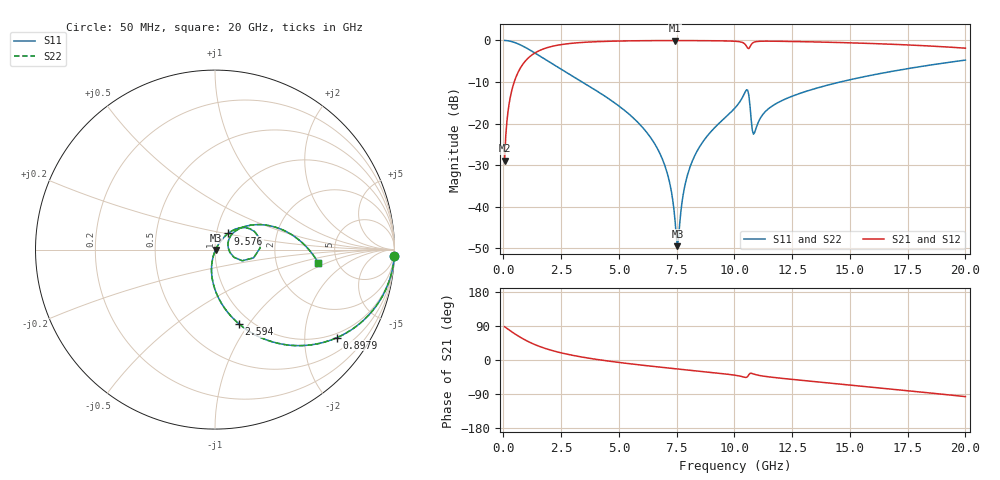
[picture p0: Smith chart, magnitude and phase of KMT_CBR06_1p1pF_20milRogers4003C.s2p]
! Data measured by Modelithics Inc. support@modelithics.com 813-866-6335
! KEMET CBR0603 1.1pF, Pad Width= 0.851mm, Pad Length= 0.64mm, Pad Gap= 0.62mm, 20mil Rogers 4003C substrate Data, January 2022
# hz S ma R 50
! 2 Port Network Data from SP1.SP block
! freq  magS11  angS11  magS21  angS21  magS12  angS12  magS22  angS22
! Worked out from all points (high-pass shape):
!   401 points, 50 MHz to 20 GHz, reference 50 ohm
!   highest |S21| = -0.03 dB at 7.431 GHz (marker M1); lowest = -29.0 dB at 50 MHz (marker M2)
!   |S21| within 3 dB of the highest: 1.358 GHz to end of sweep
!   lowest |S11| = -49.5 dB at 7.531 GHz (marker M3), VSWR 1.01, Z = 50.3 - j0.159 ohm
!   |S11| at or under -10 dB: 3.411 GHz to 14.58 GHz (11.17 GHz wide, 124 % of centre)
!   |S22| runs from -49.5 to 0.0 dB; largest |S21 - S12| = 0
!   S11 on the Smith chart (normalised r, x): 50 MHz: 1, -52; 897.9 MHz: 0.87, -2.86; 2.594 GHz: 0.88, -0.90; 9.576 GHz: 1.14, +0.21; 20 GHz: 3.57, -0.79
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5e7  0.9994 -2.2  0.03565 87.8  0.03565 87.8  0.9994 -2.2
1.99625e8  0.9899 -8.7  0.1411 81.2  0.1411 81.2  0.9899 -8.7
3.4925e8  0.9701 -15.1  0.2421 74.8  0.2421 74.8  0.9701 -15.1
8.97875e8  0.8384 -35.8  0.5439 54.1  0.5439 54.1  0.8384 -35.8
1.695875e9  0.6186 -57.0  0.7839 32.8  0.7839 32.8  0.6186 -57.0
2.593625e9  0.4338 -72.2  0.8987 17.5  0.8987 17.5  0.4338 -72.2
3.391625e9  0.3186 -81.7  0.9453 7.9  0.9453 7.9  0.3186 -81.7
5.53625e9  0.1227 -99.1  0.9896 -10.4  0.9896 -10.4  0.1227 -99.1
6.73325e9  0.04595 -104.7  0.9956 -18.6  0.9956 -18.6  0.04595 -104.7
7.182125e9  0.02011 -102.2  0.9963 -21.4  0.9963 -21.4  0.02011 -102.2
7.4315e9  0.006686 -83.4  0.9964 -23.0  0.9964 -23.0  0.006686 -83.4
7.53125e9  0.003339 -28.2  0.9964 -23.6  0.9964 -23.6  0.003339 -28.2
7.880375e9  0.01926 53.9  0.9961 -25.8  0.9961 -25.8  0.01926 53.9
8.179625e9  0.03544 56.6  0.9955 -27.7  0.9955 -27.7  0.03544 56.6
9.576125e9  0.1164 50.7  0.9874 -36.6  0.9874 -36.6  0.1164 50.7
1.0025e10  0.1541 46.1  0.9776 -40.2  0.9776 -40.2  0.1541 46.1
1.052375e10  0.2547 15.3  0.8512 -45.7  0.8512 -45.7  0.2547 15.3
1.087288e10  0.07764 21.6  0.9579 -37.8  0.9579 -37.8  0.07764 21.6
1.157112e10  0.1579 42.1  0.9794 -45.1  0.9794 -45.1  0.1579 42.1
1.336662e10  0.2571 32.5  0.961 -56.4  0.961 -56.4  0.2571 32.5
1.670825e10  0.419 13.0  0.902 -76.2  0.902 -76.2  0.419 13.0
2e10  0.5799 -7.3  0.8071 -96.6  0.8071 -96.6  0.5799 -7.3
